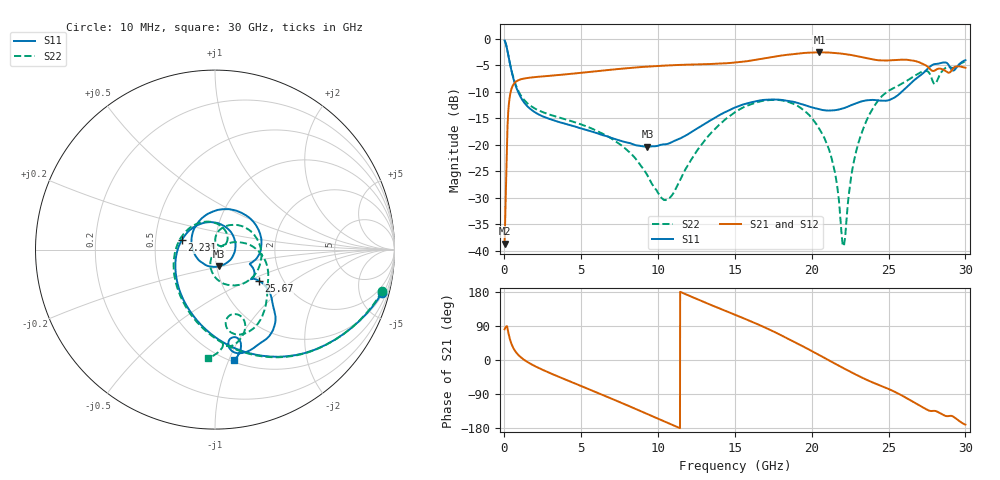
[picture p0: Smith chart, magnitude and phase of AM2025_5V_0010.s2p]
!Keysight Technologies,N5245B,MY58422270,A.16.20.02
!Date: Tuesday, July 14, 2026 01:02:38
!Correction: S11(C  2-Port  )
!S21(C  2-Port  )
!S12(C  2-Port  )
!S22(C  2-Port  )
!S2P File: Measurements: S11, S21, S12, S22:
# Hz S  dB  R 50
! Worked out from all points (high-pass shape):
!   3201 points, 10 MHz to 30 GHz, reference 50 ohm
!   highest |S21| = -2.59 dB at 20.5 GHz (marker M1); lowest = -38.7 dB at 10 MHz (marker M2)
!   |S21| within 3 dB of the highest: 7.965 GHz to 27.65 GHz (19.68 GHz wide, 111 % of centre); 29.22 GHz to end of sweep
!   lowest |S11| = -20.4 dB at 9.307 GHz (marker M3), VSWR 1.21, Z = 51.3 - j9.65 ohm
!   |S11| at or under -10 dB: 877.9 MHz to 25.87 GHz (24.99 GHz wide, 187 % of centre)
!   |S22| runs from -39.2 to -0.4 dB; largest |S21 - S12| = 0.0083
!   S11 on the Smith chart (normalised r, x): 10 MHz: 1.21, -7.57; 2.231 GHz: 0.68, +0.08; 25.67 GHz: 1.51, -0.57; 30 GHz: 0.52, -1.05
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1e7  -0.35 -14.7  -38.66 81.2  -35.00 80.6  -0.36 -14.0
2.630406e8  -3.34 -61.3  -13.17 70.4  -13.16 70.5  -3.32 -61.5
4.411062e8  -5.88 -86.6  -9.63 44.2  -9.64 44.1  -5.80 -86.8
9.659312e8  -10.55 -132.4  -7.78 10.8  -7.78 10.8  -10.24 -131.5
2.231134e9  -14.32 163.8  -7.20 -21.1  -7.20 -21.1  -13.57 170.8
5.014581e9  -16.97 70.6  -6.45 -69.1  -6.44 -69.0  -16.22 96.6
9.3069e9  -20.39 -77.0  -5.29 -142.7  -5.28 -142.7  -25.80 25.5
1.000979e10  -20.20 -105.4  -5.17 -155.0  -5.17 -155.0  -29.20 35.3
1.084389e10  -19.61 -139.7  -5.04 -169.7  -5.04 -169.7  -29.77 71.0
1.5005e10  -13.00 84.1  -4.52 119.4  -4.52 119.4  -13.90 39.5
1.776033e10  -11.50 17.2  -3.32 70.4  -3.32 70.4  -11.57 -26.5
2.000958e10  -12.98 -16.8  -2.63 23.4  -2.62 23.4  -15.01 -82.1
2.049692e10  -13.32 -20.0  -2.59 12.8  -2.59 12.7  -17.03 -93.5
2.143411e10  -13.54 -22.7  -2.69 -7.9  -2.69 -7.8  -24.30 -112.7
2.207139e10  -13.14 -23.8  -2.89 -21.7  -2.89 -21.7  -39.12 -43.9
2.259622e10  -12.53 -26.0  -3.11 -32.8  -3.12 -32.9  -25.47 27.7
2.308356e10  -12.00 -29.2  -3.38 -42.8  -3.38 -42.9  -19.24 22.1
2.500479e10  -11.63 -38.0  -4.11 -76.5  -4.11 -76.6  -9.84 -23.1
2.567019e10  -10.52 -35.4  -4.00 -89.4  -4.00 -89.4  -8.83 -36.0
2.756331e10  -5.62 -50.1  -5.35 -132.4  -5.35 -132.4  -6.22 -75.5
2.807877e10  -4.78 -62.2  -5.89 -134.9  -5.89 -135.0  -8.40 -71.4
3e10  -4.09 -80.1  -5.51 -170.4  -5.50 -170.6  -4.33 -93.9
